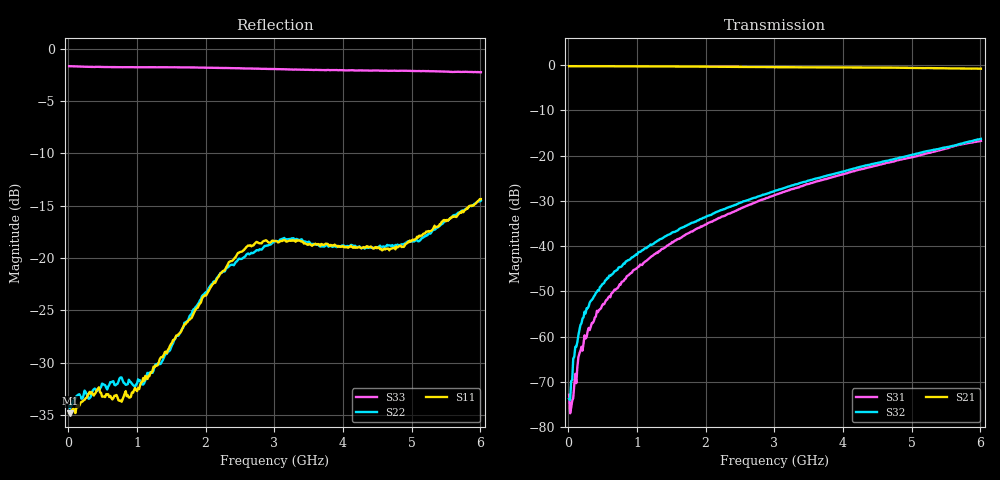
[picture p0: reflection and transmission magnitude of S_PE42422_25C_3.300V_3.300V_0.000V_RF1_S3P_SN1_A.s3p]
! Device ID: PE42422
! Serial: 1
! Insertion: A
! Temp: 25C
! VDD: 3.300
! Control_Hi: 3.300
! Control_Lo: 0.000
! Logic State: RF1
! Port 1: RFC
! Port 2: RF1
! Port 3: RF2
! ThroughPath:2-1
! V1 = 3.30
! V2 = 0.00
! V3 = 0.00
! V4 = 0.00
! IDD: 1.013644e-04
#  Hz  S  RI  R  50
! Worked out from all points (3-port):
!   401 points, 10 MHz to 6.01 GHz, reference 50 ohm
!   strongest paths, dB at 10 MHz, 1.51 GHz, 3.01 GHz, 4.51 GHz, 6.01 GHz:
!     S21: -0.2, -0.3, -0.4, -0.5, -0.8
!     S32: -73.7, -37.0, -27.7, -21.6, -16.3
!     S31: -72.8, -39.1, -28.7, -22.1, -16.7
!   lowest |S11| = -34.8 dB at 25 MHz (marker M1), VSWR 1.04, Z = 51.8 + j0.0546 ohm
!   |S11| at or under -10 dB: start of sweep to end of sweep
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1e7  0.0182 -4.32e-05  0.9758 -0.00238  0.000177 -3e-05
     0.9758 -0.00158  0.0196 -0.000777  0.000111 -6.41e-05
     -0.000171 0.000151  0.000194 -6.9e-05  -0.8245 0.00273
2.5e7  0.0181 0.000527  0.9756 -0.0039  4.94e-05 0.000124
       0.9753 -0.00404  0.0191 0.00074  6.73e-05 0.000209
       -1.99e-05 0.000141  5.57e-05 0.000191  -0.8242 0.00593
1e8  0.0181 0.0018  0.9748 -0.0148  -2.11e-05 0.000291
     0.9748 -0.015  0.0212 0.00191  6.24e-05 0.000778
     -3.19e-05 0.000387  1.08e-05 0.000771  -0.822 0.0211
2.05e8  0.0203 0.00364  0.9741 -0.0306  -0.000194 0.000831
        0.9738 -0.0303  0.0211 0.00343  3.01e-05 0.0015
        -0.000133 0.000688  -1.3e-05 0.00159  -0.8193 0.0406
6.1e8  0.0219 -0.00157  0.9692 -0.0881  -0.0013 0.00268
       0.969 -0.0882  0.0255 -0.00208  -0.000701 0.00465
       -0.00126 0.00242  -0.000762 0.00463  -0.8083 0.1121
1.54e9  0.00927 -0.0396  0.9434 -0.2197  -0.00708 0.00886
        0.9433 -0.2194  0.0123 -0.0386  -0.00507 0.0134
        -0.007 0.00893  -0.00522 0.0134  -0.7773 0.2441
2.47e9  -0.0281 -0.102  0.8942 -0.3432  -0.0161 0.0195
        0.8935 -0.3424  -0.0191 -0.096  -0.0118 0.027
        -0.016 0.0195  -0.0117 0.027  -0.7218 0.3596
3.01e9  -0.0392 -0.114  0.8601 -0.4098  -0.0223 0.029
        0.8602 -0.4103  -0.0385 -0.1139  -0.0155 0.0378
        -0.0225 0.0291  -0.0154 0.0381  -0.6709 0.4342
4.705e9  -0.0849 -0.0712  0.7107 -0.6141  -0.0381 0.0764
         0.7122 -0.6135  -0.054 -0.1004  -0.0218 0.0873
         -0.0378 0.0763  -0.0218 0.0873  -0.4397 0.6489
6.01e9  -0.188 -0.0352  0.5343 -0.7423  -0.0338 0.1416
        0.5324 -0.7439  -0.1205 -0.1443  -0.00861 0.1533
        -0.0333 0.1419  -0.00822 0.1532  -0.2912 0.7141
